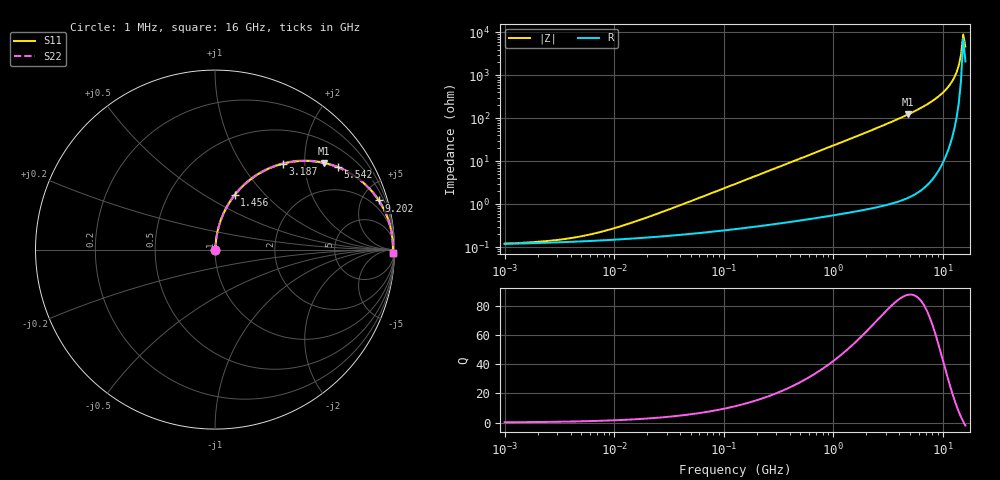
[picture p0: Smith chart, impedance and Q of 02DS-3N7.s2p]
# MHz S MA R 50
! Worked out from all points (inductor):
!   211 points, 1 MHz to 16 GHz, reference 50 ohm
!   read as one part in series: L = 3.7 nH near 22.98 MHz
!   highest Q = 87.8 at 4.826 GHz (marker M1), where L = 4.1 nH
!   self-resonance near 15.28 GHz
!   S11 on the Smith chart (normalised r, x): 1 MHz: 1.00, +0.00; 1.456 GHz: 1.01, +0.68; 3.187 GHz: 1.02, +1.55; 5.542 GHz: 1.03, +2.96; 9.202 GHz: 1.13, +6.62; 16 GHz: 43, -84
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1  0.001211 11.0  0.9988 -0.0  0.9988 -0.0  0.001211 11.0
2.51416  0.001398 24.6  0.9987 -0.0  0.9987 -0.0  0.001398 24.6
5.25662  0.001834 41.6  0.9986 -0.1  0.9986 -0.1  0.001834 41.6
10.4954  0.002862 58.2  0.9985 -0.1  0.9985 -0.1  0.002862 58.2
26.3872  0.006373 73.6  0.9982 -0.4  0.9982 -0.4  0.006373 73.6
132.458  0.03081 83.3  0.9969 -1.8  0.9969 -1.8  0.03081 83.3
333.021  0.07703 82.9  0.9935 -4.4  0.9935 -4.4  0.07703 82.9
664.915  0.1524 79.5  0.9837 -8.8  0.9837 -8.8  0.1524 79.5
1455.79  0.3213 70.2  0.9409 -18.7  0.9409 -18.7  0.3213 70.2
2204.33  0.4607 61.7  0.8806 -27.4  0.8806 -27.4  0.4607 61.7
3187.38  0.6083 51.8  0.786 -37.5  0.786 -37.5  0.6083 51.8
4826.25  0.7749 38.6  0.6233 -50.8  0.6233 -50.8  0.7749 38.6
5542.03  0.8239 33.9  0.5573 -55.5  0.5573 -55.5  0.8239 33.9
7307.8  0.9049 24.4  0.4136 -64.8  0.4136 -64.8  0.9049 24.4
9202.05  0.9523 16.7  0.2875 -72.2  0.2875 -72.2  0.9523 16.7
11587.3  0.9809 9.2  0.1597 -78.5  0.1597 -78.5  0.9809 9.2
12706.4  0.9871 6.2  0.1087 -80.1  0.1087 -80.1  0.9871 6.2
13305.8  0.9892 4.8  0.08328 -80.2  0.08328 -80.2  0.9892 4.8
13933.5  0.9906 3.3  0.058 -79.0  0.058 -79.0  0.9906 3.3
14590.9  0.9912 1.8  0.03307 -73.6  0.03307 -73.6  0.9912 1.8
15279.2  0.9911 0.4  0.01104 -36.3  0.01104 -36.3  0.9911 0.4
16000  0.9903 -1.1  0.02104 62.2  0.02104 62.2  0.9903 -1.1
